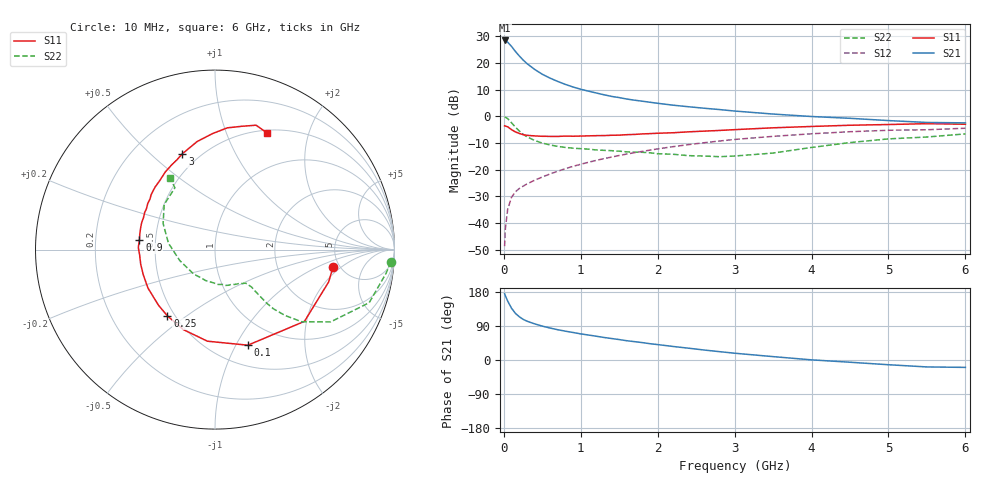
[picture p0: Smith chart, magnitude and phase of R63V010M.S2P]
! SIEMENS Small Signal Semiconductors
! BFR193
! Si NPN RF Bipolar Junction Transistor in SOT23
! VCE = 3 V  IC = 10 mA
! Common Emitter S-Parameters:  May  1996
# GHz  S  MA  R  50
!  f  S11  S21  S12  S22
! GHz  MAG  ANG  MAG  ANG  MAG  ANG  MAG  ANG
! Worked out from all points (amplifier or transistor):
!   36 points, 10 MHz to 6 GHz, reference 50 ohm
!   highest |S21| = 28.4 dB at 10 MHz (marker M1)
!   |S21| within 3 dB of that: start of sweep to 120.5 MHz
!   unconditionally stable (mu >= 1): 728.6 MHz to 1.886 GHz
!   at 250 MHz: K = 0.65, MSG = 23.7 dB, |S12| = -26.2 dB
!   at 1.4 GHz: K = 1.04, MAG = 10.1 dB, |S12| = -15.2 dB
!   at 6 GHz: K = 0.95, MSG = 1.0 dB, |S12| = -4.4 dB
!   lowest NFmin = 1.30 dB at 450 MHz
!   S11 on the Smith chart (normalised r, x): 10 MHz: 4.42, -1.52; 100 MHz: 0.72, -1.12; 250 MHz: 0.46, -0.43; 900 MHz: 0.41, +0.05; 3 GHz: 0.41, +0.64; 6 GHz: 0.53, +1.40
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0.01  0.665 -8.3  26.45 174.9  0.0037 86.9  0.9824 -4.0
0.02  0.6583 -15.9  26.15 169.5  0.0079 86.2  0.9621 -7.9
0.05  0.639 -38.7  24.52 155.5  0.0182 73.7  0.9086 -19.0
0.1  0.5633 -71.0  20.47 136.6  0.0306 63.6  0.76 -32.0
0.15  0.5121 -94.7  16.46 123.2  0.0385 57.6  0.6279 -39.8
0.2  0.4795 -111.5  13.61 114.3  0.0444 55.7  0.5337 -43.3
0.25  0.4547 -125.6  11.41 107.4  0.0492 55.4  0.4628 -45.4
0.3  0.4418 -135.5  9.776 102.5  0.0542 56.3  0.4148 -46.0
0.4  0.4306 -150.1  7.59 95.4  0.0636 57.5  0.3538 -46.0
0.5  0.4235 -160.9  6.151 89.4  0.0731 59.7  0.3161 -46.0
0.6  0.4218 -169.0  5.21 84.4  0.0834 60.9  0.2916 -45.7
0.7  0.4209 -175.7  4.518 79.9  0.0937 61.9  0.2743 -46.4
0.9  0.4248 172.9  3.549 72.6  0.1157 62.6  0.2536 -47.6
1.1  0.4314 164.1  2.969 65.9  0.1379 62.9  0.2431 -51.3
1.3  0.4363 156.0  2.544 59.5  0.1615 62.2  0.2309 -55.1
1.6  0.4541 145.6  2.109 50.8  0.1972 60.2  0.2161 -63.5
2.2  0.4934 128.3  1.621 35.7  0.2708 54.2  0.1951 -84.8
3  0.5641 108.8  1.259 17.9  0.3695 43.5  0.1807 -131.0
3.5  0.6107 99.3  1.105 8.9  0.4223 35.9  0.2054 -162.6
4.5  0.6819 84.2  0.92 -5.9  0.5159 20.9  0.3231 153.4
5.5  0.7299 71.7  0.769 -18.3  0.5615 5.3  0.4105 123.0
6  0.7122 66.1  0.756 -19.5  0.5996 0.8  0.4697 122.0
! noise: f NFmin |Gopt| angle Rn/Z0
0.45  1.3  0.22  143  0.11
0.9  1.3  0.34  160  0.11
1.8  2.05  0.54  -153  0.14
